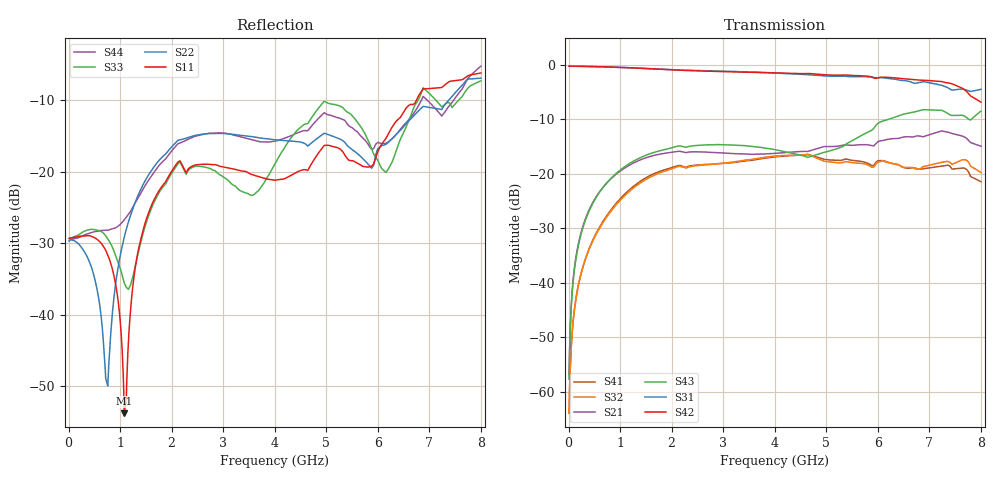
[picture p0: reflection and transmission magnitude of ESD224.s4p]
! Created Thu Mar  1 16:08:46 2018
# hz S ma R 50
! 4 Port Network Data from SP1.SP block
! freq  magS11  angS11  magS12  angS12  magS13  angS13  magS14  angS14
!  magS21  angS21  magS22  angS22  magS23  angS23  magS24  angS24
!  magS31  angS31  magS32  angS32  magS33  angS33  magS34  angS34
!  magS41  angS41  magS42  angS42  magS43  angS43  magS44  angS44
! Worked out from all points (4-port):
!   800 points, 10 MHz to 8 GHz, reference 50 ohm
!   strongest paths, dB at 10 MHz, 2.01 GHz, 4.01 GHz, 6.01 GHz, 8 GHz:
!     S42: -0.3, -1.0, -1.5, -2.4, -6.9
!     S31: -0.3, -0.9, -1.5, -2.4, -4.5
!     S43: -57.6, -15.2, -15.6, -10.7, -8.5
!     S21: -57.6, -16.1, -16.3, -14.1, -15.0
!     S32: -63.9, -19.1, -16.8, -17.8, -19.8
!     S41: -63.8, -18.9, -16.9, -17.6, -21.5
!   lowest |S11| = -53.8 dB at 1.08 GHz (marker M1), VSWR 1.00, Z = 49.9 - j0.179 ohm
!   |S11| at or under -10 dB: start of sweep to 6.75 GHz
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1e7  0.03418 -0.4  0.001238 152.4  0.9666 -0.1  0.0006799 151.9
     0.001312 -15.4  0.03282 4.9  0.0009008 -25.9  0.9684 -0.4
     0.9665 -0.2  0.0006367 71.1  0.03409 1.9  0.001252 -167.5
     0.0006429 -155.1  0.9668 -0.5  0.001324 -179.5  0.03272 7.4
2e8  0.03525 -6.6  0.02413 61.5  0.964 -3.4  0.01009 86.2
     0.02405 61.3  0.03111 -18.6  0.01006 84.0  0.9646 -3.1
     0.9639 -3.4  0.009977 83.6  0.03625 41.3  0.02318 109.1
     0.01008 85.3  0.9646 -3.1  0.02311 109.2  0.03458 28.4
7.4e8  0.02712 -47.8  0.08204 -12.6  0.9512 -11.8  0.04123 74.0
       0.08211 -12.7  0.003373 -142.2  0.04028 69.5  0.9518 -11.1
       0.9512 -11.8  0.04019 69.6  0.03472 115.9  0.08221 162.1
       0.04119 74.0  0.9519 -11.1  0.08227 162.1  0.03895 74.5
1.08e9  0.002046 -118.6  0.112 -58.6  0.9395 -16.6  0.06429 65.0
        0.1121 -58.6  0.03478 92.6  0.06226 61.7  0.9394 -15.7
        0.9394 -16.7  0.06232 61.6  0.01664 117.5  0.115 -164.7
        0.06437 64.9  0.9396 -15.8  0.1152 -164.6  0.04596 74.6
2.12e9  0.1165 -36.3  0.1603 161.4  0.8931 -31.5  0.1184 37.4
        0.1602 161.3  0.1653 -26.8  0.1161 39.7  0.8896 -29.1
        0.8929 -31.5  0.116 39.7  0.113 132.4  0.1789 -64.0
        0.1184 37.3  0.8899 -29.1  0.1791 -64.0  0.1564 135.2
6.41e9  0.2344 -17.2  0.2108 -103.7  0.7224 -92.1  0.1198 -0.7
        0.211 -103.7  0.1905 -8.9  0.1205 8.3  0.7486 -78.7
        0.722 -92.1  0.1202 8.3  0.1585 6.7  0.3388 103.7
        0.1197 -0.8  0.7484 -78.7  0.3392 103.7  0.1915 30.1
8e9  0.4886 -137.8  0.1781 50.2  0.5926 -108.4  0.08632 -91.6
     0.1785 50.1  0.4501 -124.7  0.1028 -99.3  0.4539 -97.6
     0.5928 -108.5  0.1026 -99.4  0.4309 54.1  0.3741 -63.8
     0.08447 -91.8  0.4526 -97.6  0.3742 -64.0  0.5454 48.5
